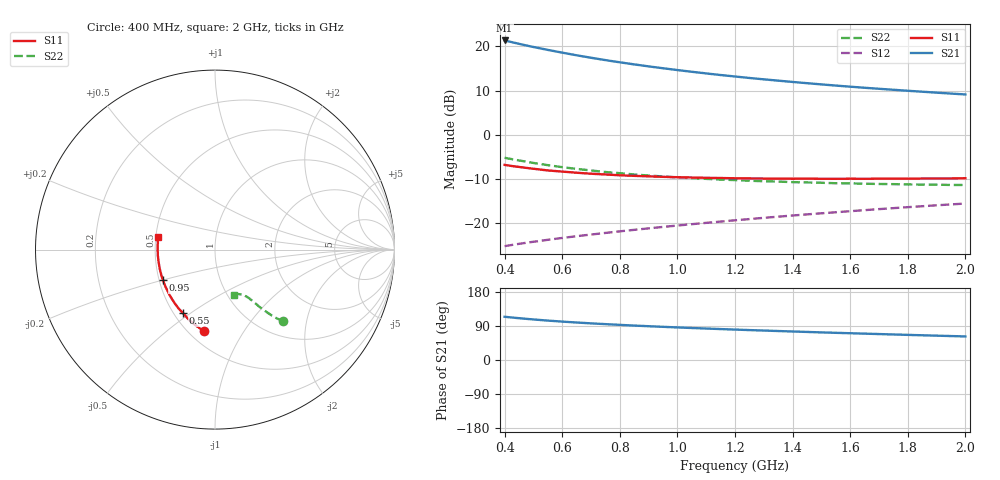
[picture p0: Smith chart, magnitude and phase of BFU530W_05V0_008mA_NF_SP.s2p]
! Filename:  P:\Prog\Test\Noise\ATS_data\Testdata_Net\06 Compressed Noise after Statistics\BFU530W_APM2013_09_A05_05p0V_008mA_NF_CM01_D.sf
! Date/Time: Tue 26/Mar/2013 18:06:05
! BFU530W_APM2013_09_A05_05p0V_1to25mA_NF_CM01_Bias5_R.sf
! Noise Parameter Data File
! BFU530W_APM2013_09_A05_05p0V_1to25mA_NF_CM01
! Date/time: Thu Mar 21 20:31:54 2013
! VAR V_out= 5.000000
! VAR I_out= 7.990000
! VAR V_in= 0.825500
! VAR I_in= 0.083905
! Device data file deembeded for feedlines and parallel
! Original file: \06 Compressed Noise after Statistics\BFU530W_APM2013_09_A05_05p0V_008mA_NF_CM01_R.sf
! Feed-files: PR019V01_070313_Feed1.s2p, PR019V01_070313_Feed2.s2p
! Parallel-file: PR019V01_070313_Par.s2p
# MHz S MA R 50
!  Freq-MHz  S11-mag  S11-arg  S21-mag  S21-arg  S12-mag  S12-arg  S22-mag  S22-arg
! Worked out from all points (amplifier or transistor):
!   37 points, 400 MHz to 2 GHz, reference 50 ohm
!   highest |S21| = 21.3 dB at 400 MHz (marker M1)
!   |S21| within 3 dB of that: start of sweep to 620.9 MHz
!   unconditionally stable (mu >= 1): 1.478 GHz to end of sweep
!   at 500 MHz: K = 0.66, MSG = 22.0 dB, |S12| = -24.1 dB
!   at 1.1 GHz: K = 0.95, MSG = 16.9 dB, |S12| = -19.9 dB
!   at 2 GHz: K = 1.02, MAG = 11.4 dB, |S12| = -15.5 dB
!   lowest NFmin = 0.68 dB at 433 MHz
!   S11 on the Smith chart (normalised r, x): 400 MHz: 0.59, -0.68; 550 MHz: 0.56, -0.47; 950 MHz: 0.52, -0.20; 2 GHz: 0.51, +0.08
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400  0.4585 -97.6  11.63 114.1  0.05547 57.5  0.5517 -46.4
420  0.4482 -100.5  11.23 112.5  0.05689 57.3  0.5361 -47.1
433  0.4414 -102.3  10.97 111.6  0.0578 57.2  0.5263 -47.6
460  0.4307 -105.9  10.48 109.7  0.0596 57.1  0.5081 -48.3
500  0.4147 -111.1  9.817 107.0  0.06218 57.0  0.4824 -49.3
550  0.3969 -116.6  9.103 104.0  0.06544 57.2  0.4555 -50.3
600  0.3853 -122.0  8.475 101.3  0.06868 57.4  0.4321 -51.1
650  0.374 -126.7  7.912 98.9  0.07187 57.7  0.4134 -51.8
700  0.3646 -131.3  7.42 96.7  0.07504 58.1  0.3964 -52.4
750  0.3574 -135.3  6.981 94.6  0.07824 58.5  0.3813 -52.8
800  0.3499 -139.3  6.593 92.7  0.08154 58.9  0.3696 -53.4
850  0.3449 -143.0  6.244 90.9  0.08478 59.2  0.3575 -53.8
950  0.3362 -149.4  5.649 87.5  0.09147 60.0  0.3396 -54.6
1050  0.3304 -155.3  5.154 84.5  0.0982 60.6  0.3248 -55.4
1150  0.326 -160.7  4.739 81.6  0.1051 61.1  0.3129 -56.2
1200  0.3238 -163.1  4.56 80.3  0.1087 61.4  0.3089 -56.8
1250  0.3225 -165.6  4.389 79.0  0.1122 61.5  0.3038 -57.2
1350  0.3208 -169.8  4.093 76.5  0.1194 61.9  0.2969 -58.2
1500  0.3196 -176.0  3.714 72.8  0.1303 62.1  0.2881 -60.1
1650  0.3194 178.5  3.402 69.6  0.1414 62.3  0.2812 -61.8
1750  0.3204 175.2  3.229 67.4  0.149 62.2  0.2781 -63.1
2000  0.3244 167.3  2.861 62.2  0.168 61.9  0.2722 -66.9
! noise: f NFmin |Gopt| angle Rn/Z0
400  0.6865  0.05465  106.5  0.086
460  0.708  0.05824  119.6  0.0823
600  0.7256  0.0565  119.7  0.086
800  0.7731  0.09475  133.9  0.0797
1000  0.7988  0.1189  140.1  0.0781
1200  0.8177  0.144  147.5  0.0764
1400  0.855  0.1635  156.3  0.074
1600  0.8552  0.1927  163.4  0.0706
1800  0.9067  0.194  171.4  0.0723
2000  0.9323  0.2377  177.1  0.0678
